PROGRAM MAIN_CM

VAR CONSTANT
	cInitSpectrum 	: ST_CM_MagnitudeSpectrum_InitPars := (	nFFT_Length := cFFTLength, 
															nWindowLength := cWindowLength, 
															bTransformToDecibel:= FALSE, 
															eWindowType := E_CM_WindowType.eCM_HannWindow, 
															eScalingType := E_CM_ScalingType.eCM_PeakAmplitude);
															
	// change eScalingType to E_CM_ScalingType.eCM_PeakAmplitude if max of spectrum has to be the amplitude value of a sine-wave
														
END_VAR

VAR	
	fbSpectrum			: FB_CMA_MagnitudeSpectrum :=(	stInitPars := cInitSpectrum, 
														nOwnID := eID_Spectrum, 
														aDestIDs := [eID_Sink] );
	
	fbErrHist			: FB_HRErrHist; // error monitoring
END_VAR

// Call spectrum call
fbSpectrum.Call();
IF fbSpectrum.bError THEN
	fbErrHist.AddError(bErr:=TRUE, hrErrCode:=fbSpectrum.hrErrorCode, sErrSource:='MAIN_CM.fbSpectrum'); // error monitoring
	// ToDo: if error
END_IF

END_PROGRAM
